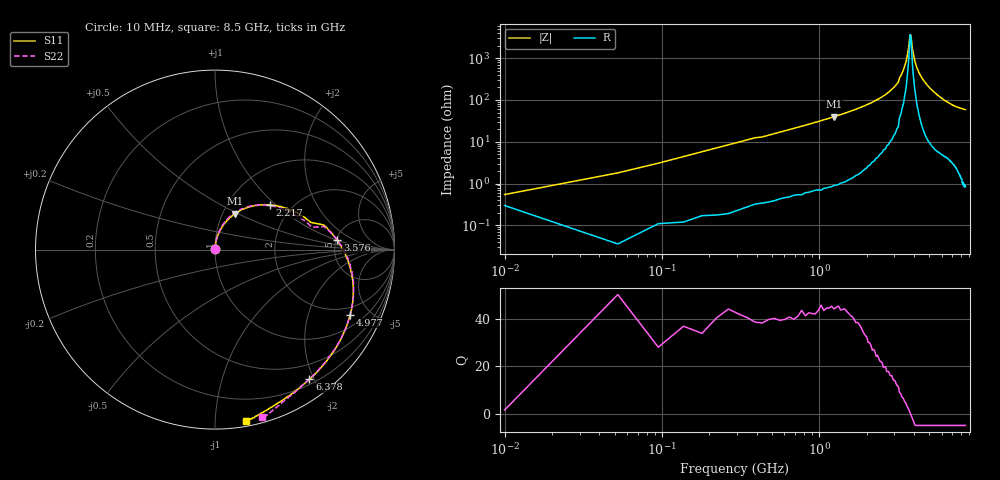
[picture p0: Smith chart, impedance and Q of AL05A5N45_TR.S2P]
!AVX Corporation
!PN: AL05A5N45*TR
!Description: Air Core Inductor, 5.45nH, 5 Turns
!Agilent Technologies,E5071C,MY46102230,A.09.54
!Date: Mon Sep 03 16:09:49 2012
!Data & Calibration Information:
!Freq	S11:SOLT2(ON)	S21:SOLT2(ON)	S12:SOLT2(ON)	S22:SOLT2(ON)
# Hz S dB R 50
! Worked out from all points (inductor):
!   201 points, 10 MHz to 8.5 GHz, reference 50 ohm
!   read as 1/Y11, port 2 shorted: L = 5.14 nH near 52.45 MHz
!   highest Q = 44.9 at 1.241 GHz (marker M1), where L = 5.09 nH
!   self-resonance near 3.788 GHz
!   S11 on the Smith chart (normalised r, x): 10 MHz: 1.00, +0.01; 2.217 GHz: 1.54, +0.91; 3.576 GHz: 5.10, +1.02; 4.977 GHz: 1.57, -3.77; 6.378 GHz: 0.27, -1.93; 8.5 GHz: 0.04, -1.20
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1e7  -51.37 74.1  -0.01 -0.3  -0.08 -0.4  -50.19 76.1
5.245e7  -37.87 85.1  -0.01 -1.3  0.01 -1.4  -37.77 86.2
9.49e7  -33.00 84.8  -0.02 -2.2  -0.01 -2.2  -33.02 84.7
1.3735e8  -29.93 84.1  -0.02 -3.2  -0.00 -3.2  -29.84 84.1
1.798e8  -27.62 82.6  -0.02 -4.2  -0.01 -4.2  -27.55 83.2
2.647e8  -24.47 81.2  -0.04 -6.1  -0.02 -6.2  -24.45 82.6
3.9205e8  -21.11 78.5  -0.07 -9.1  -0.05 -9.1  -21.09 79.4
4.345e8  -21.17 77.5  -0.07 -9.7  -0.06 -9.7  -21.14 78.9
7.3165e8  -16.88 71.2  -0.15 -16.2  -0.13 -16.3  -16.85 72.8
1.24105e9  -12.73 60.4  -0.33 -27.7  -0.33 -27.7  -12.71 62.4
1.4533e9  -11.48 56.3  -0.43 -32.5  -0.43 -32.6  -11.48 57.4
2.2174e9  -8.10 39.4  -0.93 -50.4  -0.93 -50.4  -8.10 38.4
2.85415e9  -6.02 24.2  -1.52 -65.7  -1.51 -65.7  -6.03 21.7
3.19375e9  -5.11 15.8  -1.90 -74.0  -1.89 -74.1  -5.12 12.9
3.2362e9  -4.16 12.9  -2.44 -75.8  -2.44 -75.8  -4.12 11.9
3.5758e9  -3.31 4.5  -3.10 -83.6  -3.10 -83.7  -3.30 4.3
4.255e9  -2.20 -10.8  -4.48 -98.6  -4.48 -98.6  -2.21 -10.0
4.97665e9  -1.55 -25.7  -5.87 -113.9  -5.88 -113.9  -1.58 -24.9
5.6983e9  -1.20 -40.4  -7.33 -129.3  -7.33 -129.4  -1.22 -40.8
6.3775e9  -0.97 -54.0  -8.96 -142.5  -8.96 -142.5  -0.96 -54.7
7.09915e9  -0.72 -66.2  -10.90 -153.2  -10.90 -153.3  -0.65 -65.4
8.5e9  -0.27 -79.8  -14.63 -168.0  -14.65 -168.0  -0.27 -74.4
